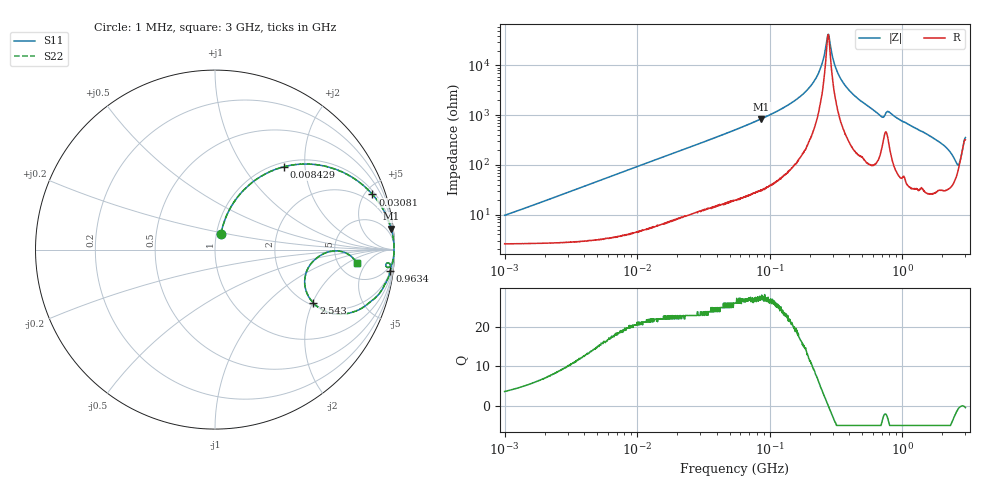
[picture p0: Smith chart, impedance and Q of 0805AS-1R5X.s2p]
!s-Parameter Generated by FASTRON Sdn. Bhd.
!FASTRON P/N : 0805AS-1R5X
!Keysight Technologies: E4991B_MY54100416_A.01.15
!Date: Mon Jun 15 12:56:54 2026
!Version  :Rev01  Mon Jun 15 12:56:54 2026
!Data & Calibration Information:
!Freq  S11  S21  S12  S22
!PortZ  Port1:50+j0  Port2:50+j0
!When reading reference impedance value at option line is always used.
! Remarks : This data is being provided solely for informational purposes.
# Hz S dB R 50
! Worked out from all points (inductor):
!   1601 points, 1 MHz to 3 GHz, reference 50 ohm
!   read as one part in series: L = 1.48 uH near 1.041 MHz
!   highest Q = 27.4 at 86.36 MHz (marker M1), where L = 1.55 uH
!   self-resonance near 275.7 MHz
!   S11 on the Smith chart (normalised r, x): 1 MHz: 1.05, +0.19; 8.429 MHz: 1.08, +1.56; 30.81 MHz: 1.24, +5.61; 963.4 MHz: 2, -16; 2.543 GHz: 2.09, -2.04; 3 GHz: 7.43, -3.08
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1000000  -20.50 69.3  -0.26 -5.2  -0.26 -5.2  -20.50 69.3
3804036  -9.74 66.4  -0.73 -18.9  -0.73 -18.9  -9.74 66.4
8429145  -4.43 50.2  -2.28 -36.9  -2.28 -36.9  -4.43 50.2
1.447069e7  -2.13 36.0  -4.62 -51.4  -4.62 -51.4  -2.13 36.0
3.080651e7  -0.63 19.3  -9.60 -68.2  -9.60 -68.2  -0.63 19.3
5.504702e7  -0.23 11.0  -14.40 -76.8  -14.40 -76.8  -0.23 11.0
8.636184e7  -0.10 6.7  -18.60 -81.2  -18.60 -81.2  -0.10 6.7
1.505037e8  -0.04 3.0  -25.50 -84.1  -25.50 -84.1  -0.04 3.0
2.083556e8  -0.02 1.4  -32.40 -83.1  -32.40 -83.1  -0.02 1.4
2.421036e8  -0.02 0.6  -38.90 -77.6  -38.90 -77.6  -0.02 0.6
2.689295e8  -0.02 0.1  -49.40 -46.5  -49.40 -46.5  -0.02 0.1
2.771263e8  -0.02 -0.0  -52.50 2.0  -52.50 2.0  -0.02 -0.0
3.204059e8  -0.02 -0.7  -38.10 78.1  -38.10 78.1  -0.02 -0.7
3.855751e8  -0.03 -1.6  -30.90 82.8  -30.90 82.8  -0.03 -1.6
6.889699e8  -0.21 -5.8  -19.80 73.8  -19.80 73.8  -0.21 -5.8
7.925923e8  -0.20 -4.7  -21.50 72.1  -21.50 72.1  -0.20 -4.7
9.633956e8  -0.14 -7.0  -18.20 79.0  -18.20 79.0  -0.14 -7.0
1.950859e9  -0.83 -19.0  -9.69 64.6  -9.69 64.6  -0.83 -19.0
2.347656e9  -2.05 -27.1  -6.63 50.5  -6.63 50.5  -2.05 -27.1
2.543347e9  -4.09 -28.5  -5.34 33.4  -5.34 33.4  -4.09 -28.5
2.783064e9  -4.52 -2.8  -7.80 4.1  -7.80 4.1  -4.52 -2.8
3e9  -2.00 -5.5  -13.00 20.1  -13.00 20.1  -2.00 -5.5
